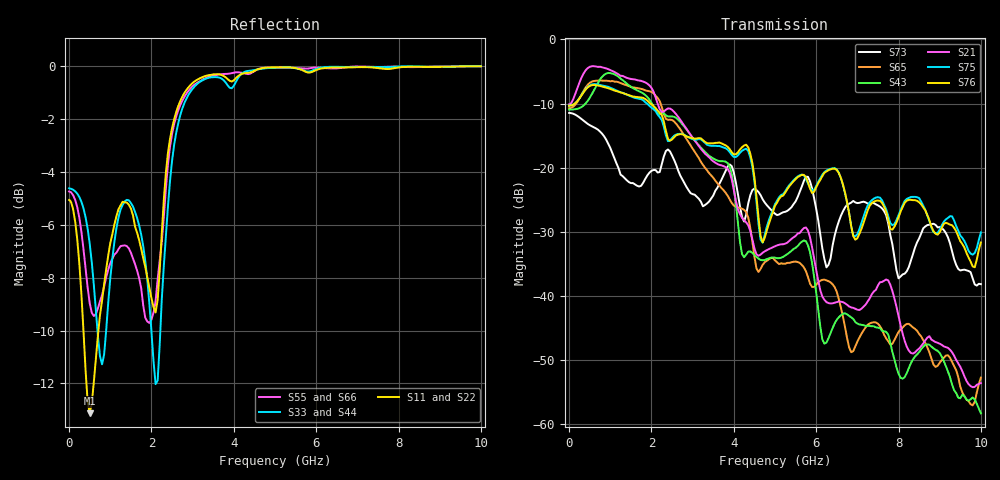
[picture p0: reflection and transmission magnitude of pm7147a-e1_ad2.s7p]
# GHz S DB R 50
! S-Parameters data
! Freq  dbS11  angS11  dbS12  angS12  dbS13  angS13  dbS14  angS14
!  dbS15  angS15  dbS16  angS16  dbS17  angS17  dbS21  angS21
!  dbS22  angS22  dbS23  angS23  dbS24  angS24  dbS25  angS25
!  dbS26  angS26  dbS27  angS27  dbS31  angS31  dbS32  angS32
!  dbS33  angS33  dbS34  angS34  dbS35  angS35  dbS36  angS36
!  dbS37  angS37  dbS41  angS41  dbS42  angS42  dbS43  angS43
!  dbS44  angS44  dbS45  angS45  dbS46  angS46  dbS47  angS47
!  dbS51  angS51  dbS52  angS52  dbS53  angS53  dbS54  angS54
!  dbS55  angS55  dbS56  angS56  dbS57  angS57  dbS61  angS61
!  dbS62  angS62  dbS63  angS63  dbS64  angS64  dbS65  angS65
!  dbS66  angS66  dbS67  angS67  dbS71  angS71  dbS72  angS72
!  dbS73  angS73  dbS74  angS74  dbS75  angS75  dbS76  angS76
!  dbS77  angS77
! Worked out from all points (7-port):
!   279 points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, 1 Hz to 10 GHz, reference 50 ohm
!   strongest paths, dB at 1 Hz, 7.943 MHz, 3.05 GHz, 6.55 GHz, 10 GHz:
!     S76: -10.3, -10.3, -15.5, -20.8, -31.7
!     S75: -10.3, -10.3, -15.6, -20.8, -30.1
!     S21: -10.1, -10.1, -15.8, -40.9, -53.6
!     S43: -10.9, -10.9, -15.8, -43.3, -58.3
!     S65: -10.7, -10.7, -17.5, -40.5, -52.8
!     S73: -11.5, -11.5, -24.2, -28.4, -38.2
!   lowest |S11| = -13.1 dB at 500 MHz (marker M1), VSWR 1.57, Z = 31.9 + j0.409 ohm
!   |S11| at or under -10 dB: 348.1 MHz to 711.8 MHz (363.6 MHz wide, 68.6 % of centre)
